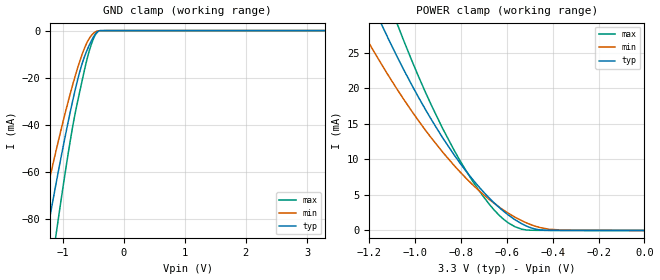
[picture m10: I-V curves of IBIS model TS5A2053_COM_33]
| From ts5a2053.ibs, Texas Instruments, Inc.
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[Model]   TS5A2053_COM_33
Model_type  Terminator
| variable   typ   min   max
C_comp   11.68pF   10.58pF   13.33pF
| C_tri-state   11.68pF   10.58pF   13.33pF
[Temperature Range]   40   100   -40
| Ambient temperature   25   85   -40
[Voltage range]   3.3   3   3.6
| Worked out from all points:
|   GND clamp passes 1 mA (typ) near -0.45 V on its own axis
|   POWER clamp passes 1 mA (typ) near -0.54 V on its own axis
[GND Clamp]
| TS5A2053_COM_33
|   Voltage   I(typ)   I(min)   I(max)
-5.5V     -821.7mA   -663.9mA   -1.071A
-1.42V    -110.6mA   -87.69mA   -146.3mA
-1.37V    -103.1mA   -81.63mA   -136.5mA
-1.265V   -87.56mA   -69.16mA   -116.3mA
-1.215V   -80.33mA   -63.35mA   -106.8mA
-1.115V   -66.2mA    -52.02mA   -88.29mA
-1.07V    -60.01mA   -47.07mA   -80.17mA
-850mV    -31.74mA   -24.55mA   -43.19mA
-725mV    -18.14mA   -13.59mA   -26.74mA
-550mV    -5.517mA   -2.868mA   -7.537mA
-415mV    -286.5uA   -95.56uA   -291uA
3.3V      586.4pA    10.98uA    4.127nA
[POWER Clamp]
| TS5A2053_COM_33
|   Voltage   I(typ)   I(min)   I(max)
-5.5V     656.7mA    519.9mA    861.4mA
-1.245V   36.08mA    28.84mA    44.33mA
-1.145V   28.87mA    23.28mA    34.87mA
-1.08V    24.53mA    19.93mA    29.2mA
-1.05V    22.62mA    18.45mA    26.71mA
-930mV    15.63mA    13.04mA    17.67mA
-830mV    10.63mA    9.141mA    11.28mA
-725mV    6.252mA    5.702mA    5.785mA
-615mV    2.722mA    2.876mA    1.594mA
-535mV    943.4uA    1.373mA    179.8uA
-455mV    76.2uA     406.7uA    17.82uA
-95.1fV   586.4pA    4.44nA     14.39nA
